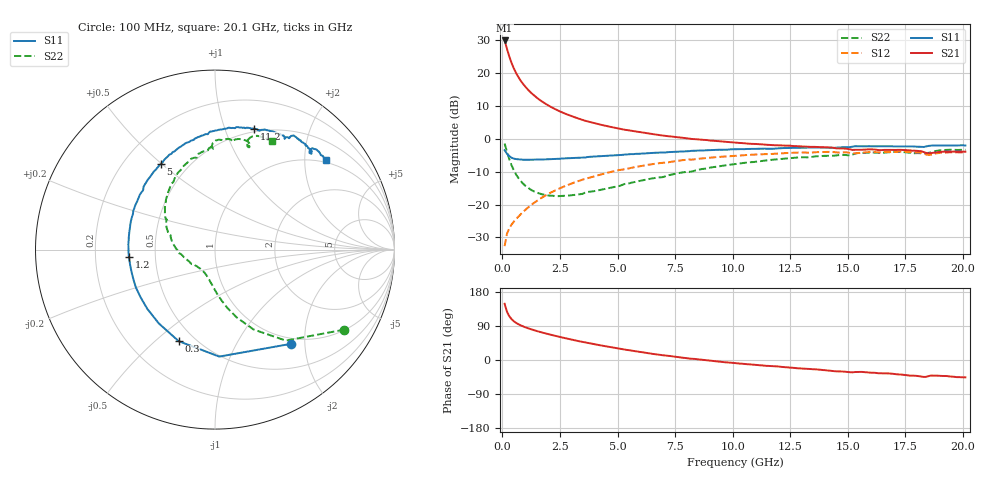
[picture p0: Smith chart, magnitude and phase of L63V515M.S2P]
!  Infineon Technologies AG
! BFR380L3 , PF131585-7, No.6, Th 09.10.01, soldered on pcb-board, measured with PP GSG850
!  Vce=3.5 V,  Ic=15.0 mA
! Common Emitter S-Parameters:  15. November 2001
#  GHz  S  MA  R  50
! f  S11  S21  S12  S22
! GHz  Mag  Ang  Mag  Ang  Mag  Ang  Mag  Ang
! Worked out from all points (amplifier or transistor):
!   201 points, 100 MHz to 20.1 GHz, reference 50 ohm
!   highest |S21| = 30.0 dB at 100 MHz (marker M1)
!   |S21| within 3 dB of that: start of sweep to 221.8 MHz
!   unconditionally stable (mu >= 1): 1.587 GHz to 4.427 GHz
!   at 3.4 GHz: K = 1.02, MAG = 8.4 dB, |S12| = -12.6 dB
!   at 10.1 GHz: K = 0.95, MSG = 2.0 dB, |S12| = -5.1 dB
!   at 20.1 GHz: K = 0.99, MSG = 0.1 dB, |S12| = -4.1 dB
!   S11 on the Smith chart (normalised r, x): 100 MHz: 0.89, -1.72; 300 MHz: 0.41, -0.60; 1.2 GHz: 0.35, -0.04; 5 GHz: 0.35, +0.50; 11.2 GHz: 0.47, +1.27; 20.1 GHz: 0.94, +2.52
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0.1  0.6737 -51.2  31.5 148.3  0.02327 67.0  0.8478 -31.7
0.2  0.5966 -87.7  23.65 127.9  0.03572 56.7  0.6421 -52.1
0.3  0.5488 -111.6  18.06 115.8  0.04355 52.8  0.4946 -64.2
0.4  0.5168 -127.3  14.36 107.9  0.04947 51.9  0.3974 -72.2
0.5  0.5013 -138.7  11.84 102.3  0.05507 53.0  0.3326 -78.0
0.6  0.4926 -147.1  10.05 98.0  0.06044 54.1  0.2868 -82.5
0.7  0.4888 -154.1  8.713 94.4  0.06565 55.4  0.2533 -86.4
0.8  0.4843 -159.5  7.686 91.4  0.0714 56.7  0.2281 -89.7
0.9  0.4815 -164.4  6.874 88.8  0.07728 57.7  0.2085 -92.6
1  0.4805 -168.4  6.225 86.3  0.08312 58.6  0.1935 -95.5
1.2  0.4814 -175.3  5.228 82.0  0.09519 59.8  0.1717 -100.6
1.6  0.4836 174.0  3.975 74.6  0.1201 60.9  0.1477 -110.0
2.1  0.492 163.7  3.078 66.7  0.1519 60.5  0.1367 -120.9
2.7  0.505 153.2  2.443 58.0  0.1899 58.7  0.1359 -133.4
3.5  0.5192 140.8  1.935 47.5  0.2406 54.9  0.1462 -146.5
5  0.5648 122.1  1.448 30.5  0.3311 46.0  0.1895 -171.9
6.8  0.6168 103.4  1.145 13.8  0.4263 34.1  0.2593 162.9
10.1  0.6937 78.5  0.8784 -8.2  0.5529 12.7  0.4139 129.1
11.2  0.7084 72.1  0.8278 -14.0  0.5825 5.6  0.4584 119.1
13.5  0.7359 60.9  0.757 -24.4  0.6237 -8.3  0.535 100.5
16.8  0.7727 48.4  0.6791 -35.5  0.6314 -24.5  0.6271 78.8
20.1  0.7924 38.9  0.6377 -45.8  0.625 -38.3  0.6846 62.2
